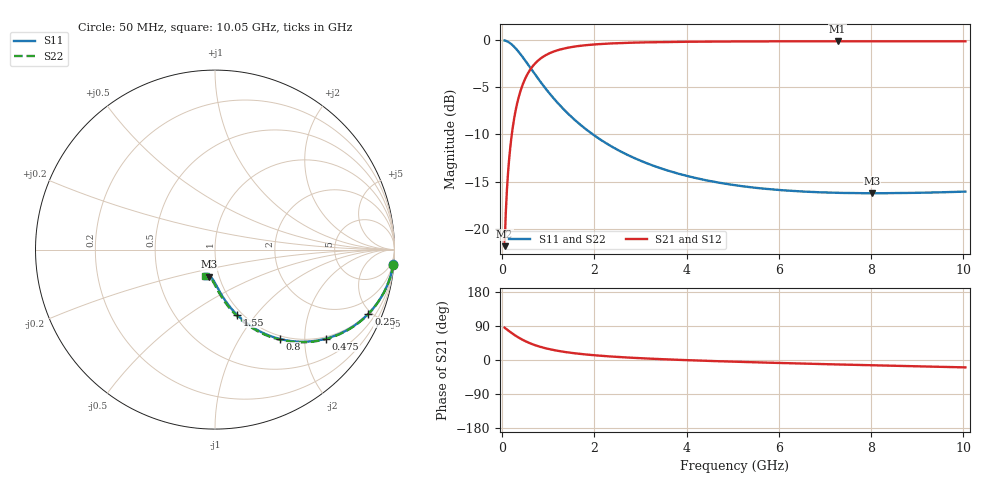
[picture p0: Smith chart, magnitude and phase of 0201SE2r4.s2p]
! AVX Thin Film Operation		Date: August 2001
! Description: Accu-P® Series, Thin Film, SMD, RF Capacitor
! Part Number: 02013J2R4ABW
! 50 MHz  -  10.05 GHz
! Serial Measurements
# mhz S db R 50
!	S11		S21		S12		S22
!	dB	Phase	dB	Phase	dB	Phase	dB	Phase
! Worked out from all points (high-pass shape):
!   401 points, 50 MHz to 10.05 GHz, reference 50 ohm
!   highest |S21| = -0.11 dB at 7.275 GHz (marker M1); lowest = -21.9 dB at 50 MHz (marker M2)
!   |S21| within 3 dB of the highest: 606.5 MHz to end of sweep
!   lowest |S11| = -16.2 dB at 8.025 GHz (marker M3), VSWR 1.36, Z = 44.8 - j13.8 ohm
!   |S11| at or under -10 dB: 1.966 GHz to end of sweep
!   |S22| runs from -16.2 to 0.0 dB; largest |S21 - S12| = 0.00011
!   S11 on the Smith chart (normalised r, x): 50 MHz: 1, -24; 250 MHz: 0.95, -4.81; 475 MHz: 0.95, -2.54; 800 MHz: 0.95, -1.52; 1.55 GHz: 0.95, -0.80; 10.05 GHz: 0.87, -0.27
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50  -0.03 -4.8  -21.85 85.2  -21.85 85.2  -0.03 -4.8
75  -0.06 -7.1  -18.37 82.9  -18.37 82.9  -0.06 -7.2
125  -0.18 -11.8  -14.04 78.2  -14.04 78.2  -0.18 -11.8
150  -0.25 -14.0  -12.54 75.9  -12.54 75.9  -0.25 -14.1
200  -0.43 -18.5  -10.22 71.5  -10.22 71.5  -0.43 -18.6
250  -0.66 -22.7  -8.52 67.2  -8.52 67.2  -0.66 -22.8
350  -1.21 -30.4  -6.15 59.5  -6.15 59.5  -1.21 -30.6
475  -2.01 -38.7  -4.32 51.1  -4.32 51.1  -2.01 -39.0
625  -3.04 -46.8  -2.98 43.0  -2.98 43.0  -3.04 -47.2
800  -4.23 -54.1  -2.06 35.6  -2.06 35.6  -4.23 -54.6
950  -5.19 -59.0  -1.57 30.7  -1.57 30.7  -5.19 -59.6
1125  -6.23 -63.6  -1.19 26.0  -1.19 26.0  -6.23 -64.3
1550  -8.36 -71.4  -0.69 18.0  -0.69 18.0  -8.36 -72.4
1725  -9.10 -73.8  -0.58 15.6  -0.58 15.6  -9.10 -74.8
2500  -11.62 -81.1  -0.32 8.1  -0.32 8.1  -11.63 -82.5
3400  -13.53 -86.4  -0.20 2.5  -0.20 2.5  -13.53 -88.2
5050  -15.38 -93.2  -0.14 -4.6  -0.14 -4.6  -15.39 -95.4
6725  -16.11 -98.5  -0.12 -10.1  -0.12 -10.1  -16.11 -100.9
7275  -16.19 -100.1  -0.12 -11.8  -0.12 -11.8  -16.19 -102.5
8025  -16.24 -102.3  -0.12 -13.9  -0.12 -13.9  -16.24 -104.7
8400  -16.23 -103.3  -0.12 -15.0  -0.12 -15.0  -16.23 -105.7
10050  -16.07 -107.8  -0.12 -19.5  -0.12 -19.5  -16.07 -110.1
